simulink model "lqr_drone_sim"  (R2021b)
settings: Solver=ode4  StartTime=0.0  StopTime=50  FixedStep=0.004  RelTol=1e-3
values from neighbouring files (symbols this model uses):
  g = 9.81    [drone_LQR_main.m]
  I = [Ix; Iy; Iz]    [drone_LQR_main.m]
  K_altitude = lqr(A_h, B_h, Q_h, R_h)    [drone_LQR_main.m]
  K_attitude = lqr(A, B, Q, R)    [drone_LQR_main.m]
  K_position = lqr(A_p, B_p, Q_p, R_p)    [drone_LQR_main.m]
  L = 0.15    [drone_LQR_main.m]    (also in bode_filter.m = 1/(s+1))
  mass = 1.7    [drone_LQR_main.m]
  n_F = 0.0088    [drone_LQR_main.m]
  n_T = 0.00001336    (= 1.336e-05)    [drone_LQR_main.m]
  pos_ref = [ pos_refx' pos_refy' pos_refz' ]    [trajplann3.m]
  t_ref = []    [trajplann3.m]
  ts = 0.004    [drone_LQR_main.m]
  vel_ref = [ vel_refx, vel_refy, vel_refz ]    [trajplann3.m]
undefined symbols (not defined in the file or in its folder): cosd, sind
libraries: simulink x6

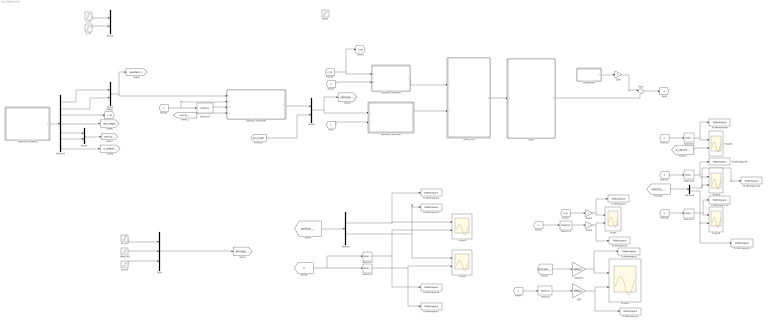
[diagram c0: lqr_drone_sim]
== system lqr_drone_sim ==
  Demux : Demux  Outputs=2
  Demux1 : Demux  Outputs=7
  Demux2 : Demux  Outputs=2
  Gain : Gain  Gain=0
  Gain2 : Gain  Gain=-1
  Gain3 : Gain  Gain=-1
  LQR : Gain  Gain=180/pi
  Mux : Mux  Commented=on  Inputs=3
  Mux1 : Mux  Inputs=2
  Mux2 : Mux  Inputs=2
  Mux3 : Mux  Inputs=2
  Mux4 : Mux  Commented=on  Inputs=2
  Scope{,1..6} (7 alike) : Scope  NumInputPorts=2
  Selector : Selector  InputPortWidth=12  IndexOptions=Index vector (dialog)  Indices=4:6  OutputSizes=1
  Selector1 : Selector  InputPortWidth=12  IndexOptions=Index vector (dialog)  Indices=6  OutputSizes=1
  Selector2 : Selector  InputPortWidth=12  IndexOptions=Index vector (dialog)  Indices=3  OutputSizes=1
  Selector3 : Selector  InputPortWidth=12  IndexOptions=Index vector (dialog)  Indices=1  OutputSizes=1
  Selector4 : Selector  InputPortWidth=12  IndexOptions=Index vector (dialog)  Indices=2  OutputSizes=1
  Selector5 : Selector  InputPortWidth=12  IndexOptions=Index vector (dialog)  Indices=9  OutputSizes=1
  Selector6 : Selector  InputPortWidth=12  IndexOptions=Index vector (dialog)  Indices=7  OutputSizes=1
  Selector7 : Selector  InputPortWidth=12  IndexOptions=Index vector (dialog)  Indices=8  OutputSizes=1
  Setpoint : Gain  Gain=180/pi
  Step2 : Step  Commented=on  After=-1  SampleTime=0
  Subsystem : Subsystem
  Sum : Sum  Inputs=|++
  To Workspace : ToWorkspace  VariableName=z_sp  SaveFormat=Timeseries  SampleTime=-1
  To Workspace1 : ToWorkspace  VariableName=z_act  SaveFormat=Timeseries  SampleTime=-1
  To Workspace10 : ToWorkspace  VariableName=y_velocity_act  SaveFormat=Timeseries  SampleTime=-1
  To Workspace12 : ToWorkspace  VariableName=x_velocity_sp  SaveFormat=Timeseries  SampleTime=-1
  To Workspace13 : ToWorkspace  VariableName=y_velocity_sp  SaveFormat=Timeseries  SampleTime=-1
  To Workspace2 : ToWorkspace  VariableName=attitude_sp  SaveFormat=Timeseries  SampleTime=-1
  To Workspace3 : ToWorkspace  VariableName=attitude_act  SaveFormat=Timeseries  SampleTime=-1
  To Workspace4 : ToWorkspace  VariableName=x_sp  SaveFormat=Timeseries  SampleTime=-1
  To Workspace5 : ToWorkspace  VariableName=y_sp  SaveFormat=Timeseries  SampleTime=-1
  To Workspace6 : ToWorkspace  VariableName=x_act  SaveFormat=Timeseries  SampleTime=-1
  To Workspace7 : ToWorkspace  VariableName=y_act  SaveFormat=Timeseries  SampleTime=-1
  To Workspace8 : ToWorkspace  VariableName=z_velocity_act  SaveFormat=Timeseries  SampleTime=-1
  To Workspace9 : ToWorkspace  VariableName=x_velocity_act  SaveFormat=Timeseries  SampleTime=-1
  Trajectory Planner1 : Subsystem
  altitude_controller : Subsystem
  attitude_controller : Subsystem
  motor_mix : Subsystem
  phi_ref : Step  Commented=on  After=20*pi/180  SampleTime=0
  plant : Subsystem
  position_controller : Subsystem
  psi_ref : Step  Commented=on  After=20*pi/180  SampleTime=0
  theta_ref : Step  Commented=on  After=20*pi/180  SampleTime=0
  x_ref : Step  Commented=on  SampleTime=0
  y_ref : Step  Commented=on  SampleTime=0
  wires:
  motor_mix/1(PWM) -> plant/1(PWM)
  psi_ref/1 -> Mux/3
  phi_ref/1 -> Mux/1
  Selector2/1 -> Gain2/1
  [x] -> Selector2/1
  [z_sp] -> Gain3/1
  [x] -> altitude_controller/2(x)
  theta_ref/1 -> Mux/2
  Gain2/1 -> To Workspace1/1, Scope/2
  Gain3/1 -> To Workspace/1, Scope/1
  [x] -> attitude_controller/2(x)
  Selector/1 -> LQR/1
  [attitude_sp] -> Setpoint/1
  Setpoint/1 -> To Workspace2/1, Scope2/1
  LQR/1 -> To Workspace3/1, Scope2/2
  [x] -> Selector/1
  attitude_controller/1(torque) -> motor_mix/2(torque)
  Selector1/1 -> position_controller/3(psi)
  [x] -> position_controller/2(x), Selector1/1
  [position_sp] -> Demux/1
  Demux/1 -> To Workspace4/1, Scope1/1
  Demux/2 -> Scope3/1, To Workspace5/1
  [x] -> Selector4/1, Selector3/1
  Selector3/1 -> Scope1/2, To Workspace6/1
  Selector4/1 -> To Workspace7/1, Scope3/2
  position_controller/1(attitude_reference) -> Mux2/1
  Trajectory Planner1/1(ref) -> Demux1/1
  Demux1/1 -> Mux1/1
  Demux1/2 -> Mux1/2
  Demux1/3 -> [z_ref]
  Demux1/4 -> [psi_angle]
  Demux1/5 -> Mux3/1
  Demux1/6 -> Mux3/2
  Demux1/7 -> [z_velocity_sp]
  Mux3/1 -> [velocity_sp]
  Selector5/1 -> To Workspace8/1, Scope4/1
  [x] -> Selector5/1
  [z_velocity_sp] -> Scope4/2
  [x] -> Selector6/1
  Selector6/1 -> To Workspace9/1, Scope5/1
  [velocity_sp] -> Demux2/1
  Demux2/1 -> To Workspace12/1, Scope5/2
  [x] -> Selector7/1
  Selector7/1 -> To Workspace10/1, Scope6/1
  Demux2/2 -> To Workspace13/1, Scope6/2
  y_ref/1 -> Mux4/2
  x_ref/1 -> Mux4/1
  Mux/1 -> [attitude_sp]
  altitude_controller/1(throttle) -> motor_mix/1(throttle)
  [z_ref] -> [z_sp], altitude_controller/1(z_ref)
  Mux1/1 -> [position_sp], position_controller/1(position_ref)
  [velocity_sp] -> position_controller/4(velocity_ref)
  [psi_angle] -> Mux2/2
  Mux2/1 -> [attitude_sp], attitude_controller/1(attitude_ref)
  Sum/1 -> [x]
  plant/1(x) -> Sum/2
  Subsystem/1(noise) -> Gain/1
  Gain/1 -> Sum/1

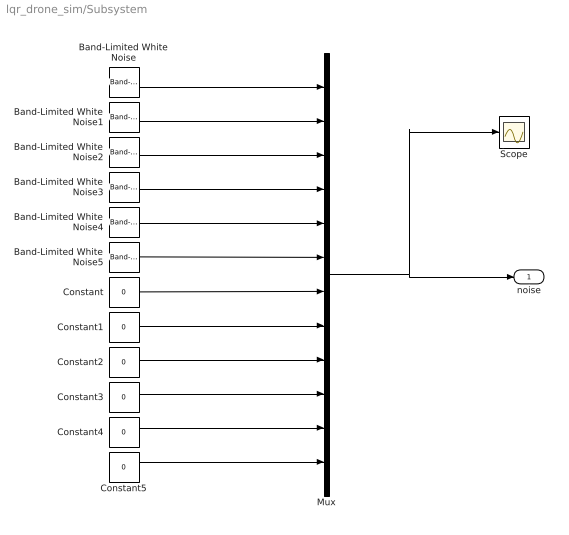
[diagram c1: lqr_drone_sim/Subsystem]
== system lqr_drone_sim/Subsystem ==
  Band-Limited White Noise : simulink/Sources/Band-Limited White Noise  Cov=0.00005  Ts=ts  seed=[11432]
  Band-Limited White Noise1 : simulink/Sources/Band-Limited White Noise  Cov=0.00005  Ts=ts  seed=[13242]
  Band-Limited White Noise2 : simulink/Sources/Band-Limited White Noise  Cov=0.00005  Ts=ts  seed=[34124]
  Band-Limited White Noise3 : simulink/Sources/Band-Limited White Noise  Cov=0.00001  Ts=ts  seed=[41123]
  Band-Limited White Noise4 : simulink/Sources/Band-Limited White Noise  Cov=0.00001  Ts=ts  seed=[32144]
  Band-Limited White Noise5 : simulink/Sources/Band-Limited White Noise  Cov=0.00001  Ts=ts  seed=[14123]
  Constant{,1..5} (6 alike) : Constant  Value=0  SampleTime=ts
  Mux : Mux  Inputs=12
  Scope : Scope
  noise : Outport
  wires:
  Band-Limited White Noise/1 -> Mux/1
  Band-Limited White Noise1/1 -> Mux/2
  Band-Limited White Noise2/1 -> Mux/3
  Band-Limited White Noise3/1 -> Mux/4
  Band-Limited White Noise4/1 -> Mux/5
  Band-Limited White Noise5/1 -> Mux/6
  Constant/1 -> Mux/7
  Constant1/1 -> Mux/8
  Constant2/1 -> Mux/9
  Constant3/1 -> Mux/10
  Constant4/1 -> Mux/11
  Constant5/1 -> Mux/12
  Mux/1 -> Scope/1, noise/1

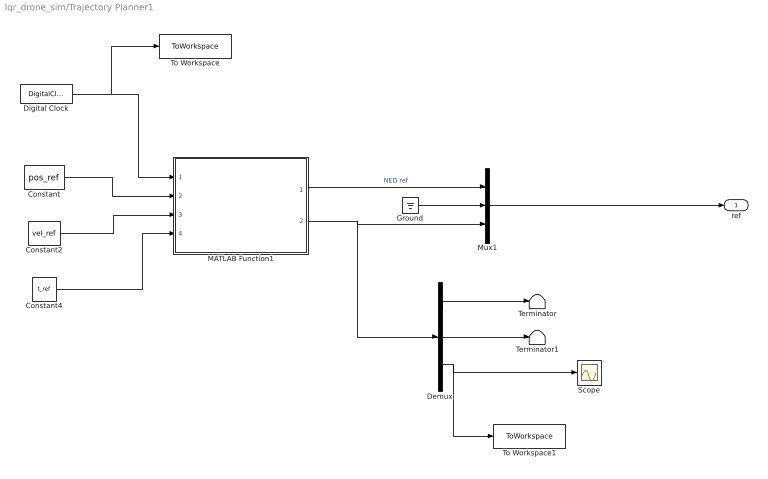
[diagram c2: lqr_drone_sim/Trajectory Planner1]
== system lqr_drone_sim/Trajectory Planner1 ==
  Constant : Constant  Value=pos_ref
  Constant2 : Constant  Value=vel_ref
  Constant4 : Constant  Value=t_ref
  Demux : Demux  Outputs=3
  Digital Clock : DigitalClock  SampleTime=0.004
  Ground : Ground
  MATLAB Function1 : MATLAB Function  TreatAsAtomicUnit=on
  Mux1 : Mux  Inputs=3
  Scope : Scope
  Terminator : Terminator
  Terminator1 : Terminator
  To Workspace : ToWorkspace  VariableName=time_sim  SaveFormat=Timeseries  SampleTime=-1
  To Workspace1 : ToWorkspace  VariableName=z_velocity_sp  SaveFormat=Timeseries  SampleTime=-1
  ref : Outport  VectorParamsAs1DForOutWhenUnconnected=off
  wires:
  MATLAB Function1/2(uvw_ref) -> Demux/1, Mux1/3
  Ground/1 -> Mux1/2
  MATLAB Function1/1(NED_ref) -> Mux1/1  "NED ref"
  Mux1/1 -> ref/1
  Constant/1 -> MATLAB Function1/2(pos_ref)
  Constant2/1 -> MATLAB Function1/3(vel_ref)
  Constant4/1 -> MATLAB Function1/4(t_ref)
  Digital Clock/1 -> To Workspace/1, MATLAB Function1/1(clk)
  Demux/1 -> Terminator/1
  Demux/2 -> Terminator1/1
  Demux/3 -> To Workspace1/1, Scope/1

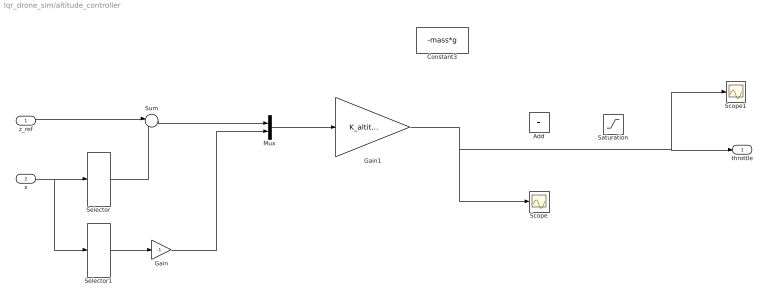
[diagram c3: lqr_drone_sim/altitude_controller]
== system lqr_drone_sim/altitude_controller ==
  z_ref : Inport
  x : Inport  Port=2
  Add : Sum  Commented=on
  Constant3 : Constant  Commented=on  Value=-mass*g
  Gain : Gain  Gain=-1
  Gain1 : Gain  Gain=K_altitude  Multiplication=Matrix(K*u) (u vector)
  Mux : Mux  Inputs=2
  Saturation : Saturate  Commented=on  UpperLimit=0  LowerLimit=-30
  Scope : Scope
  Scope1 : Scope
  Selector : Selector  InputPortWidth=12  IndexOptions=Index vector (dialog)  Indices=3  OutputSizes=1
  Selector1 : Selector  InputPortWidth=12  IndexOptions=Index vector (dialog)  Indices=9  OutputSizes=1
  Sum : Sum  Inputs=|+-
  throttle : Outport
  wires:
  x/1 -> Selector1/1, Selector/1
  z_ref/1 -> Sum/1
  Mux/1 -> Gain1/1
  Selector/1 -> Sum/2
  Gain1/1 -> Scope1/1, throttle/1, Scope/1
  Sum/1 -> Mux/1
  Selector1/1 -> Gain/1
  Gain/1 -> Mux/2

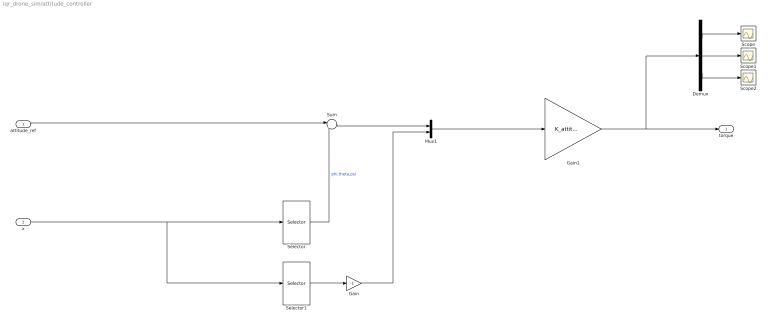
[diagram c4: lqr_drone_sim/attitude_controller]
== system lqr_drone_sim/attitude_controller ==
  attitude_ref : Inport
  x : Inport  Port=2
  Demux : Demux  Outputs=3
  Gain : Gain  Gain=-1
  Gain1 : Gain  Gain=K_attitude  Multiplication=Matrix(K*u) (u vector)
  Mux1 : Mux  Inputs=2
  Scope : Scope
  Scope1 : Scope
  Scope2 : Scope
  Selector : Selector  InputPortWidth=12  IndexOptions=Index vector (dialog)  Indices=[4,5,6]  OutputSizes=1
  Selector1 : Selector  InputPortWidth=12  IndexOptions=Index vector (dialog)  Indices=[10,11,12]  OutputSizes=1
  Sum : Sum  Inputs=|+-
  torque : Outport
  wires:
  Gain1/1 -> Demux/1, torque/1
  Gain/1 -> Mux1/2
  Selector1/1 -> Gain/1
  x/1 -> Selector1/1, Selector/1
  Selector/1 -> Sum/2  "phi,theta,psi"
  attitude_ref/1 -> Sum/1
  Sum/1 -> Mux1/1
  Mux1/1 -> Gain1/1
  Demux/1 -> Scope/1
  Demux/2 -> Scope1/1
  Demux/3 -> Scope2/1

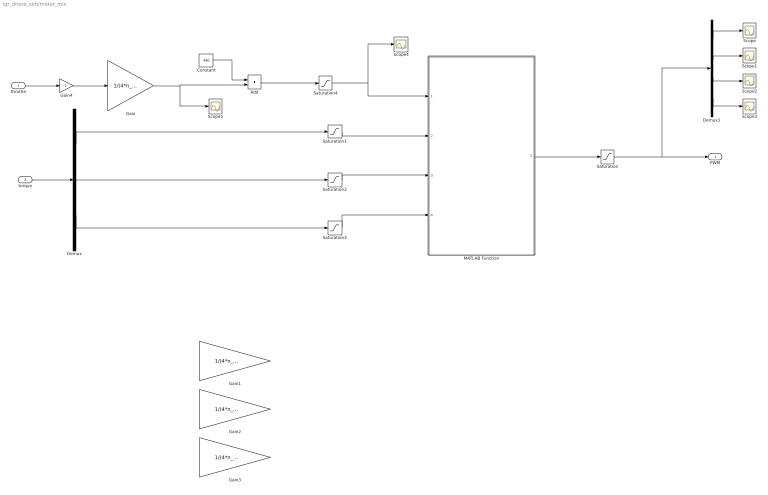
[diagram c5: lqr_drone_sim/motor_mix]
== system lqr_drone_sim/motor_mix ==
  throttle : Inport
  torque : Inport  Port=2
  Add : Sum
  Constant : Constant  Value=480
  Demux : Demux  Outputs=3
  Demux1 : Demux
  Gain : Gain  Gain=1/(4*n_F)
  Gain1 : Gain  Commented=on  Gain=1/(4*n_F*L*sind(45))
  Gain2 : Gain  Commented=on  Gain=1/(4*n_F*L*cosd(45))
  Gain3 : Gain  Commented=on  Gain=1/(4*n_T)
  Gain4 : Gain  Gain=-1
  MATLAB Function : MATLAB Function  TreatAsAtomicUnit=on
  Saturation : Saturate  UpperLimit=2000  LowerLimit=1000
  Saturation1 : Saturate  UpperLimit=300  LowerLimit=-300
  Saturation2 : Saturate  UpperLimit=300  LowerLimit=-300
  Saturation3 : Saturate  UpperLimit=300  LowerLimit=-300
  Saturation4 : Saturate  UpperLimit=800  LowerLimit=0
  Scope{,1..5} (6 alike) : Scope
  PWM : Outport
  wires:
  MATLAB Function/1(PWM) -> Saturation/1
  Saturation/1 -> Demux1/1, PWM/1
  Demux1/1 -> Scope/1
  Demux1/2 -> Scope1/1
  Demux1/3 -> Scope2/1
  Demux1/4 -> Scope3/1
  torque/1 -> Demux/1
  Saturation1/1 -> MATLAB Function/2(roll_cmd)
  Saturation2/1 -> MATLAB Function/3(pitch_cmd)
  Saturation3/1 -> MATLAB Function/4(yaw_cmd)
  Gain4/1 -> Gain/1
  throttle/1 -> Gain4/1
  Saturation4/1 -> Scope4/1, MATLAB Function/1(throttle_cmd)
  Demux/1 -> Saturation1/1
  Demux/2 -> Saturation2/1
  Demux/3 -> Saturation3/1
  Constant/1 -> Add/1
  Add/1 -> Saturation4/1
  Gain/1 -> Scope5/1, Add/2

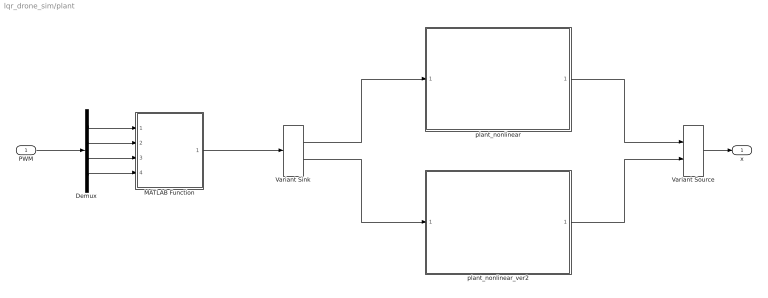
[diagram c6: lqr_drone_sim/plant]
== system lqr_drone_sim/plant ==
  PWM : Inport
  Demux : Demux
  MATLAB Function : MATLAB Function  TreatAsAtomicUnit=on
  Variant Sink : VariantSink
  Variant Source : VariantSource
  plant_nonlinear : Subsystem
  plant_nonlinear_ver2 : Subsystem
  x : Outport
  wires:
  plant_nonlinear/1(x) -> Variant Source/1
  Variant Sink/2 -> plant_nonlinear_ver2/1("u ")
  Variant Source/1 -> x/1
  plant_nonlinear_ver2/1(x) -> Variant Source/2
  Variant Sink/1 -> plant_nonlinear/1("u ")
  MATLAB Function/1(u) -> Variant Sink/1
  Demux/1 -> MATLAB Function/1(PWM_1)
  Demux/2 -> MATLAB Function/2(PWM_2)
  Demux/3 -> MATLAB Function/3(PWM_3)
  Demux/4 -> MATLAB Function/4(PWM_4)
  PWM/1 -> Demux/1

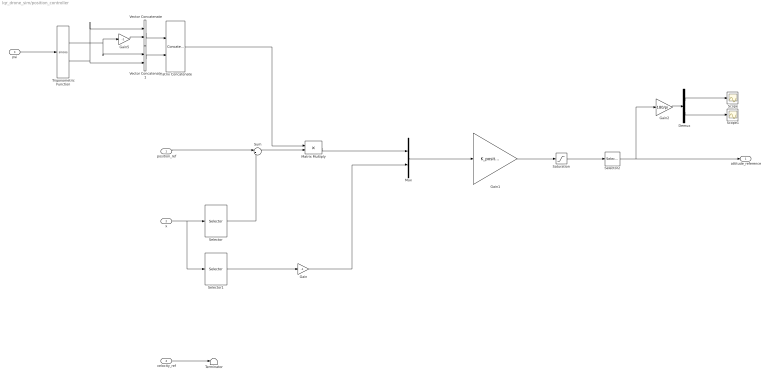
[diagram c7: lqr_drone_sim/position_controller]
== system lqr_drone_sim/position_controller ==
  position_ref : Inport
  x : Inport  Port=2
  psi : Inport  Port=3
  velocity_ref : Inport  Port=4
  Demux : Demux  Outputs=2
  Gain : Gain  Gain=-1
  Gain1 : Gain  Gain=K_position  Multiplication=Matrix(K*u) (u vector)
  Gain2 : Gain  Gain=180/pi
  Gain5 : Gain  Gain=-1
  Matrix Concatenate : Concatenate  Mode=Multidimensional array  ConcatenateDimension=2
  Matrix Multiply : Product  Multiplication=Matrix(*)
  Mux : Mux  Inputs=2
  Saturation : Saturate  UpperLimit=30*pi/180  LowerLimit=-30*pi/180
  Scope : Scope
  Scope1 : Scope
  Selector : Selector  InputPortWidth=12  IndexOptions=Index vector (dialog)  Indices=1:2  OutputSizes=1
  Selector1 : Selector  InputPortWidth=12  IndexOptions=Index vector (dialog)  Indices=7:8  OutputSizes=1
  Selector2 : Selector  InputPortWidth=2  IndexOptions=Index vector (dialog)  Indices=[2,1]  OutputSizes=1
  Sum : Sum  Inputs=|+-
  Terminator : Terminator
  Trigonometric Function : Trigonometry  Operator=sincos
  Vector Concatenate : Concatenate
  Vector Concatenate1 : Concatenate
  attitude_reference : Outport
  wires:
  Trigonometric Function/2 -> Vector Concatenate1/2, Vector Concatenate/1
  Vector Concatenate/1 -> Matrix Concatenate/1
  Trigonometric Function/1 -> Gain5/1, Vector Concatenate1/1
  Vector Concatenate1/1 -> Matrix Concatenate/2
  Gain5/1 -> Vector Concatenate/2
  psi/1 -> Trigonometric Function/1
  x/1 -> Selector1/1, Selector/1
  Selector/1 -> Sum/2
  Sum/1 -> Matrix Multiply/2
  Matrix Concatenate/1 -> Matrix Multiply/1
  Matrix Multiply/1 -> Mux/1
  Mux/1 -> Gain1/1
  Gain1/1 -> Saturation/1
  Saturation/1 -> Selector2/1
  Selector2/1 -> Gain2/1, attitude_reference/1
  position_ref/1 -> Sum/1
  Demux/1 -> Scope/1
  Demux/2 -> Scope1/1
  Gain2/1 -> Demux/1
  Gain/1 -> Mux/2
  velocity_ref/1 -> Terminator/1
  Selector1/1 -> Gain/1

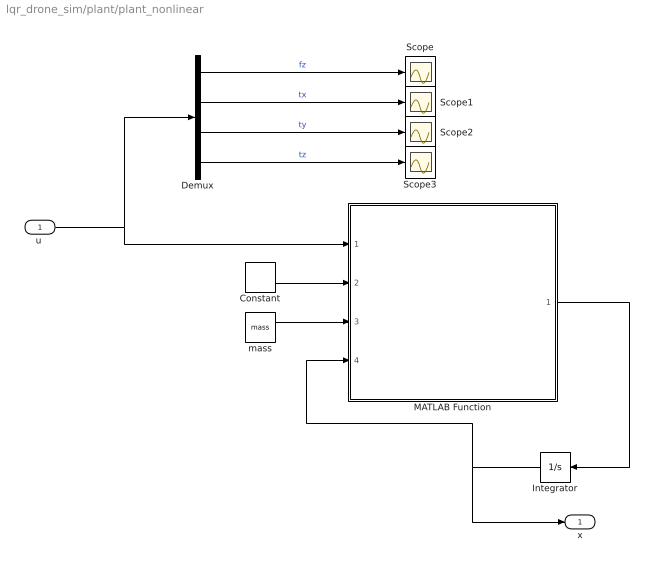
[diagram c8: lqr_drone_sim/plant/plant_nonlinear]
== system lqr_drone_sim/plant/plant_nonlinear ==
  "u " : Inport
  Constant : Constant  Value=I
  Demux : Demux
  Integrator : Integrator
  MATLAB Function : MATLAB Function  TreatAsAtomicUnit=on
  Scope{,1..3} (4 alike) : Scope
  mass : Constant  Value=mass
  x : Outport  VectorParamsAs1DForOutWhenUnconnected=off
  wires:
  mass/1 -> MATLAB Function/3(mass)
  MATLAB Function/1(xdot) -> Integrator/1
  Constant/1 -> MATLAB Function/2(I)
  Integrator/1 -> MATLAB Function/4(x), x/1
  Demux/2 -> Scope1/1  "tx"
  "u "/1 -> MATLAB Function/1(u), Demux/1
  Demux/1 -> Scope/1  "fz"
  Demux/4 -> Scope3/1  "tz"
  Demux/3 -> Scope2/1  "ty"

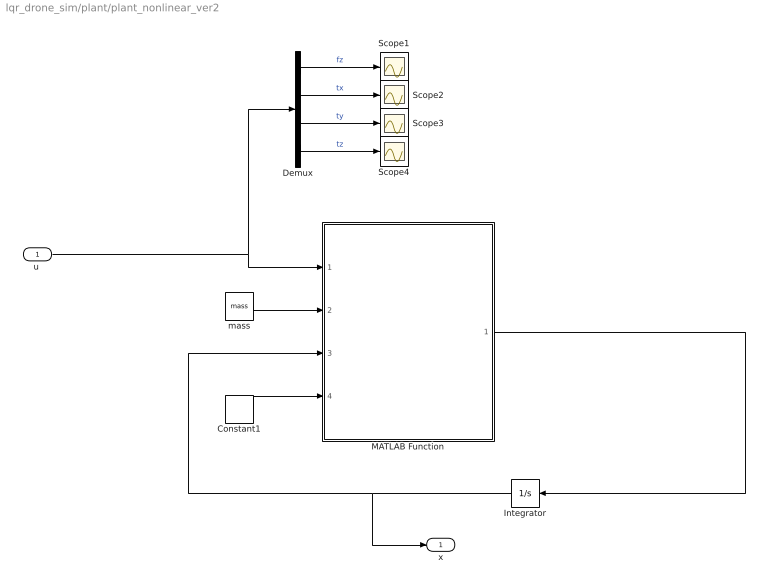
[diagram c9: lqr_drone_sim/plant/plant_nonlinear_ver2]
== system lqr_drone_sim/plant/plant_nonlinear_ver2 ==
  "u " : Inport
  Constant1 : Constant  Value=I
  Demux : Demux
  Integrator : Integrator
  MATLAB Function : MATLAB Function  TreatAsAtomicUnit=on
  Scope{1..4} (4 alike) : Scope
  mass : Constant  Value=mass
  x : Outport  VectorParamsAs1DForOutWhenUnconnected=off
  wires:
  "u "/1 -> MATLAB Function/1(u), Demux/1
  Demux/1 -> Scope1/1  "fz"
  Demux/3 -> Scope3/1  "ty"
  Demux/2 -> Scope2/1  "tx"
  Demux/4 -> Scope4/1  "tz"
  Integrator/1 -> x/1, MATLAB Function/3(x)
  mass/1 -> MATLAB Function/2(mass)
  MATLAB Function/1(xdot) -> Integrator/1
  Constant1/1 -> MATLAB Function/4(I)

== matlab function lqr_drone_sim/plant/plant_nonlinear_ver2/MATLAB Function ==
function xdot = quadrotor_dynamics(u,mass,x,I)

Ix = I(1);
Iy = I(2);
Iz = I(3);

gravity = 9.81;

phi = x(4);
theta = x(5);
psi = x(6);
U_i = x(7);
V_i = x(8);
W_i = x(9);
p = x(10);
q = x(11);
r = x(12);

%% state space representation xdot = f + g*u

f = [U_i;
     V_i;
     W_i;
     p + q*sin(phi)*tan(theta) + r*cos(phi)*tan(theta);
     q*cos(phi) - r*sin(phi);
     q*sin(phi)/cos(theta) + r*cos(phi)/cos(theta);
     0;
     0;
     gravity;
     (Iy - Iz)/Ix*q*r;
     (Iz - Ix)/Iy*p*r;
     (Ix - Iy)/Iz*p*q];


g = [0 0 0 0;
     0 0 0 0;
     0 0 0 0;
     0 0 0 0;
     0 0 0 0;
     0 0 0 0;
     (cos(phi)*sin(theta)*cos(psi) + sin(phi)*sin(psi))/mass 0 0 0;
     (cos(phi)*sin(theta)*sin(psi) - sin(phi)*cos(psi))/mass 0 0 0;
     cos(phi)*cos(theta)/mass 0 0 0;
     0 1/Ix 0 0;
     0 0 1/Iy 0;
     0 0 0 1/Iz];

xdot = f + g*u;


end

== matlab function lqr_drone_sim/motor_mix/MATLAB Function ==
function PWM = motor_mix(throttle_cmd, roll_cmd, pitch_cmd, yaw_cmd)

idel = 1000;

PWM_1 = (throttle_cmd + idel) + roll_cmd + pitch_cmd - yaw_cmd;
PWM_2 = (throttle_cmd + idel) - roll_cmd + pitch_cmd + yaw_cmd;
PWM_3 = (throttle_cmd + idel) - roll_cmd - pitch_cmd - yaw_cmd;
PWM_4 = (throttle_cmd + idel) + roll_cmd - pitch_cmd + yaw_cmd;

PWM = [PWM_1, PWM_2, PWM_3, PWM_4]';

end

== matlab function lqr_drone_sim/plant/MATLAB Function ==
function u = fcn(PWM_1, PWM_2, PWM_3, PWM_4)

L = 0.15;
n_F = 0.0088;
n_T = 0.00001336;


% thrust 

T1 = n_F*PWM_1 - 8.8085;
if T1 < 0
    T1 = 0;
end

T2 = n_F*PWM_2 - 8.8085;
if T2 < 0
    T2 = 0;
end

T3 = n_F*PWM_3 - 8.8085;
if T3 < 0
    T3 = 0;
end

T4 = n_F*PWM_4 - 8.8085;
if T4 < 0
    T4 = 0;
end


u = zeros(4,1);
u(1) = -(T1 + T2 + T3 + T4);
u(2) = (T1 + T4 - T2 - T3)*L*sind(45);
u(3) = (T1 + T2 - T3 - T4)*L*sind(45);

u(4) = -1*(n_T*PWM_1 - 0.0134) + (n_T*PWM_2 - 0.0134) - (n_T*PWM_3 - 0.0134) + (n_T*PWM_4 - 0.0134);

end

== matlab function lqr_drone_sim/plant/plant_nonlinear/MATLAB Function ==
function xdot = quadrotor_dynamics(u,I,mass,x)

ph = x(4);
th = x(5);
ps = x(6);
U = x(7);
V = x(8);
W = x(9);
p = x(10);
q = x(11);
r = x(12);
% Rotation from body to NED

% ph th and ps are in radians

            
Rb_ned = [ cos(th)*cos(ps), cos(th)*sin(ps), -sin(th)
            -cos(ph)*sin(ps) + sin(ph)*sin(th)*cos(ps), cos(ph)...
                *cos(ps) + sin(ph)*sin(th)*sin(ps), sin(ph)*cos(th)
            sin(ph)*sin(ps) + cos(ph)*sin(th)*cos(ps), -sin(ph)...
            *cos(ps) + cos(ph)*sin(th)*sin(ps), cos(ph)*cos(th) ];


% Constants linked to Inertia Moments

Ix = I(1);
Iy = I(2);
Iz = I(3);

% Non-linear plant in the form x_dot = f(x) + g(x)*u


f = [ Rb_ned'*x(7:9)
        p + tan(th)*(q*sin(ph) + r*cos(ph))
        q*cos(ph) - r*sin(ph)
        1/cos(th)*(q*sin(ph) + r*cos(ph))
        r*V - q*W - 9.81*sin(th)
        -r*U + p*W + 9.81*sin(ph)*cos(th)
        q*U - p*V + 9.81*cos(ph)*cos(th)
        (Iy - Iz)/Ix*q*r
        (Iz - Ix)/Iy*p*r
        (Ix - Iy)/Iz*p*q];

g = zeros(12,4);
g(9,1) = 1/mass;
g(10,2) = 1/Ix;
g(11,3) = 1/Iy;
g(12,4) = 1/Iz;

xdot = f + g*u;
end

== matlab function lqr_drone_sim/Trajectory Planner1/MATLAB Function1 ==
function [ NED_ref, uvw_ref ] = trajectoryPlanner(clk,pos_ref,vel_ref,t_ref)

currTime = find(clk >= t_ref);
NED_ref = pos_ref(currTime(end),:);
uvw_ref = vel_ref(currTime(end),:);
end
